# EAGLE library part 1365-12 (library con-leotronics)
DUAL ROW STRAIGHT HEADER 1364 SERIES. 1.27mm x 1.27mm. Without Fixing Post. SMT Source: http://www.leotronics.co.uk/Conexcon/Data%20Sheets/sec.%20A/1364ing.pdf
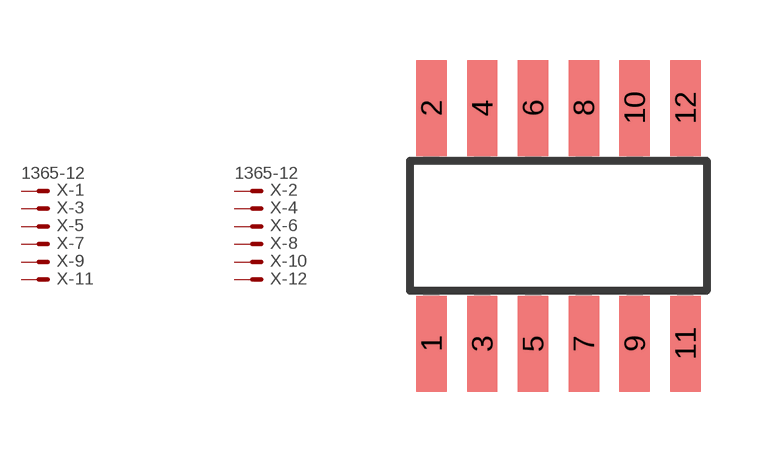
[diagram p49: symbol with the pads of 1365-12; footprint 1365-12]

Designator prefix X; gates -1=MVAL -2=MVAL -3=M -4=M -5=M -6=M -7=M -8=M -9=M -10=M -11=M -12=M

## 1365-12 (OC_FARNELL: unknown; OC_NEWARK: unknown)  [1365-12]
1  -1:S  pas
2  -2:S  pas
3  -3:S  pas
4  -4:S  pas
5  -5:S  pas
6  -6:S  pas
7  -7:S  pas
8  -8:S  pas
9  -9:S  pas
10  -10:S  pas
11  -11:S  pas
12  -12:S  pas

## Footprint 1365-12 (pad centres in mm)
DUAL ROW STRAIGHT HEADER 1364 SERIES. 1.27mm x 1.27mm. Without Fixing Post. SMT Source: http://www.leotronics.co.uk/Conexcon/Data%20Sheets/sec.%20A/1364ing.pdf
smd 0.76 x 2.4: 1 -3.175,-2.95; 2 -3.175,2.95; 3 -1.905,-2.95; 4 -1.905,2.95; 5 -0.635,-2.95; 6 -0.635,2.95; 7 0.635,-2.95; 8 0.635,2.95; 9 1.905,-2.95; 10 1.905,2.95; 11 3.175,-2.95; 12 3.175,2.95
